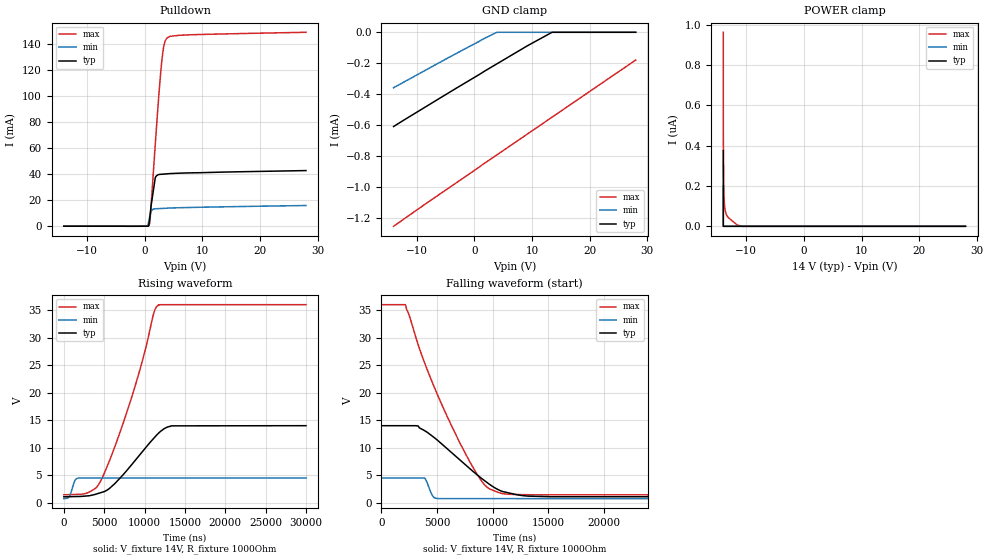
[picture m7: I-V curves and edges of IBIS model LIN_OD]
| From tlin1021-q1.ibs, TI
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|   LIN_OD
[Model]   LIN_OD
Model_type   I/O_open_drain
Polarity   Non-Inverting
Enable   Active-High
Vinl = 5.6
Vinh = 8.4
Vmeas = 7
Vref = 7
Cref = 2pF
Rref = 1000
|   typ   min   max
C_comp   12.71pF   12.14pF   13.31pF
[Voltage Range]   14   4.5   36
[Temperature Range]   25   165   -55
[Pullup Reference]   14   4.5   36
[Pulldown Reference]   0   0   0
[Power Clamp Reference]   14   4.5   36
[GND Clamp Reference]   0   0   0
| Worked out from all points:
|   slope of the pulldown table from 0 to 2.1 V, typ, clamps not added: 54.2 ohm
|   falling waveform, V_fixture 14V, R_fixture 1000Ohm: 20-80 % time 4.5us typ, 446ns min, 4.47us max; typ from 14 V to 1.07 V
|   rising waveform, V_fixture 14V, R_fixture 1000Ohm: 20-80 % time 4.52us typ, 505ns min, 4.46us max; typ from 1.07 V to 14 V
[Pulldown]
|   Voltage   I(typ)   I(min)   I(max)
-14V      -1.801uA   -1.995uA   -2.005uA
477.4mV   46.42uA    122.5uA    5.365uA
766.7mV   1.66mA     4.667mA    552uA
964.1mV   8.315mA    8.859mA    5.503mA
1.348V    21.97mA    12.73mA    29.55mA
1.86V     37.23mA    13.37mA    62.7mA
2.504V    39.71mA    13.53mA    102mA
2.929V    39.88mA    13.63mA    123.9mA
3.38V     40.03mA    13.73mA    139mA
3.983V    40.23mA    13.88mA    144.8mA
7.96V     40.95mA    14.39mA    146.9mA
28V       42.71mA    15.89mA    148.9mA
[GND Clamp]
|   Voltage   I(typ)   I(min)   I(max)
-14V      -609uA     -358.5uA   -1.254mA
-3.45V    -368.7uA   -143.3uA   -981.1uA
3.944V    -203.4uA   -82.86nA   -791.5uA
9.265V    -86.02uA   0A         -656uA
13.49V    0A         0A         -548.5uA
28V       0A         0A         -179.2uA
[POWER Clamp]
|   Voltage   I(typ)   I(min)   I(max)
-14V      376.4nA    200.2nA    962.6nA
-14V      0A         0A         595.8nA
-14V      0A         0A         568.5nA
-13.99V   0A         0A         477.5nA
-13.98V   0A         0A         388.5nA
-13.94V   0A         0A         245.7nA
-13.92V   0A         0A         192.5nA
-13.83V   0A         0A         120nA
-13.67V   0A         0A         77.97nA
-13.31V   0A         0A         49.03nA
-11.58V   0A         0A         6.384nA
28V       0A         0A         0A
[Ramp]
R_load = 1000
|   typ   min   max
dV/dt_r   7.75463/4.50162e-06   2.26078/4.9156e-07   20.7366/4.45976e-06
dV/dt_f   7.75468/4.49336e-06   2.2608/4.42529e-07   20.7368/4.46777e-06
[Falling Waveform]
V_fixture = 14V
V_fixture_min = 4.5V
V_fixture_max = 36V
R_fixture = 1000Ohm
C_fixture = 0F
|   Time   V(typ)   V(min)   V(max)
0s        14V        4.5V       36V
2.175us   14V        4.5V       35.92V
3.884us   13.1V      4.456V     25.44V
4.648us   11.99V     1.14V      21.54V
5.525us   10.51V     747.6mV    17.43V
7.982us   6.152V     746mV      7.354V
9.588us   3.549V     745mV      2.68V
10.86us   2.067V     744.2mV    1.671V
13.19us   1.199V     742.7mV    1.455V
30us      1.075V     732mV      1.438V
[Rising Waveform]
V_fixture = 14V
V_fixture_min = 4.5V
V_fixture_max = 36V
R_fixture = 1000Ohm
C_fixture = 0F
|   Time   V(typ)   V(min)   V(max)
0s        1.075V     732mV      1.438V
675.4ns   1.096V     1.141V     1.47V
1.664us   1.127V     4.444V     1.517V
3.686us   1.438V     4.479V     2.377V
4.75us    1.902V     4.48V      4.517V
8.19us    6.533V     4.483V     18.17V
11.13us   11.68V     4.485V     34.36V
11.62us   12.46V     4.486V     35.81V
13.29us   13.97V     4.487V     35.99V
30us      14V        4.5V       36V
